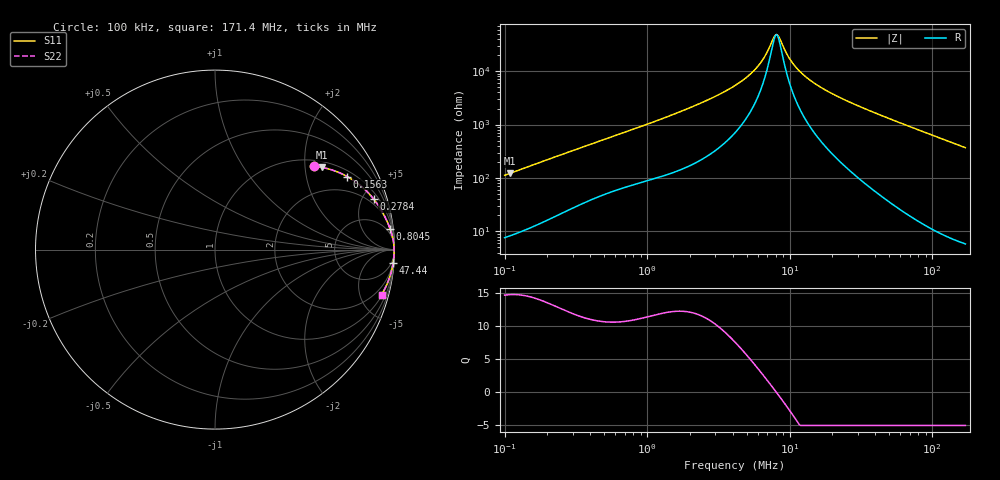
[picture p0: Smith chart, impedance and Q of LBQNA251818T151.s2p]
! LBQNA251818T151  S-PARAMETER MODEL  ( General Type )
! Model Generated by TAIYO YUDEN Corporation (http://www.ty-top.com)
! Version 1.0
! TAIYO YUDEN Control No. 191025NI43SB-FBB
! Copyright(c) 2019 TAIYO YUDEN CO.,LTD. All Rights Reserved.
! Product Description (link to TY-COMPAS)
! https://ds.yuden.co.jp/TYCOMPAS/or/detail?pn=LBQNA251818T151K&u=M
! Products Name : Inductors
! Characteristics :
!  Inductance : 150 uH , SRF(min) : 7.0 MHz , DC Resistance(max) : 4.16 Ohm
!  Rated Current : Saturation :55 mA , Temp Rise : 140 mA (20 degC)
!  Case Size : 2.5 x 1.8 / 0.098 x 0.071 [mm/inch] , Thickness : 1.8 / 0.071 [mm/inch]
!  (Conditions: Temperature = 25 degC , DC Bias Current/Voltage = 0A / 0V)
! External Node Assignments :
!  1  o---GGG---o  2
! GND o---------o GND
! Frequency Range : 0.1MHz  -  171.398534MHz  [ 402 STEP ]
# MHz S RI R 50
! Freq[MHz].  S11 Real  S11 Imag  S21 Real  S21 Imag  S12 Real  S12 Imag  S22 Real  S22 Imag
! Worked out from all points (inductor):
!   401 points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, 100 kHz to 171.4 MHz, reference 50 ohm
!   read as one part in series: L = 177 uH near 103.8 kHz
!   highest Q = 14.8 at 109.8 kHz (marker M1), where L = 178 uH
!   self-resonance near 7.943 MHz
!   S11 on the Smith chart (normalised r, x): 100 kHz: 1.15, +2.24; 156.3 kHz: 1.24, +3.47; 278.4 kHz: 1.50, +6.04; 804.5 kHz: 2, +16; 47.44 MHz: 2, -27; 171.4 MHz: 1.12, -7.39
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0.1  0.554 0.4642  0.446 -0.4642  0.446 -0.4642  0.554 0.4642
0.109755  0.5957 0.4581  0.4043 -0.4581  0.4043 -0.4581  0.5957 0.4581
0.156329  0.7369 0.4068  0.2631 -0.4068  0.2631 -0.4068  0.7369 0.4068
0.278404  0.8831 0.2829  0.1169 -0.2829  0.1169 -0.2829  0.8831 0.2829
0.348094  0.9152 0.2381  0.0848 -0.2381  0.0848 -0.2381  0.9152 0.2381
0.804492  0.975 0.117  0.025 -0.117  0.025 -0.117  0.975 0.117
1.211692  0.9867 0.0797  0.0133 -0.0797  0.0133 -0.0797  0.9867 0.0797
2.551485  0.9955 0.036  0.00451 -0.036  0.00451 -0.036  0.9955 0.036
4.140031  0.9972 0.0183  0.00275 -0.0183  0.00275 -0.0183  0.9972 0.0183
5.080878  0.9976 0.0123  0.0024 -0.0123  0.0024 -0.0123  0.9976 0.0123
6.00764  0.9978 0.00769  0.00221 -0.00769  0.00221 -0.00769  0.9978 0.00769
6.717598  0.9979 0.00476  0.00213 -0.00476  0.00213 -0.00476  0.9979 0.00476
7.796401  0.9979 0.000941  0.00206 -0.000941  0.00206 -0.000941  0.9979 0.000941
8.092155  0.998 -8.31e-06  0.00205 8.31e-06  0.00205 8.31e-06  0.998 -8.31e-06
8.399129  0.998 -0.000958  0.00204 0.000958  0.00204 0.000958  0.998 -0.000958
9.56818  0.998 -0.0043  0.00203 0.0043  0.00203 0.0043  0.998 -0.0043
10.69891  0.998 -0.00722  0.00205 0.00722  0.00205 0.00722  0.998 -0.00722
14.41119  0.9978 -0.0156  0.00221 0.0156  0.00221 0.0156  0.9978 -0.0156
22.52891  0.9971 -0.0309  0.00293 0.0309  0.00293 0.0309  0.9971 -0.0309
47.43959  0.9927 -0.0722  0.00735 0.0722  0.00735 0.0722  0.9927 -0.0722
50.16444  0.992 -0.0766  0.00802 0.0766  0.00802 0.0766  0.992 -0.0766
171.3985  0.9283 -0.2502  0.0717 0.2502  0.0717 0.2502  0.9283 -0.2502
